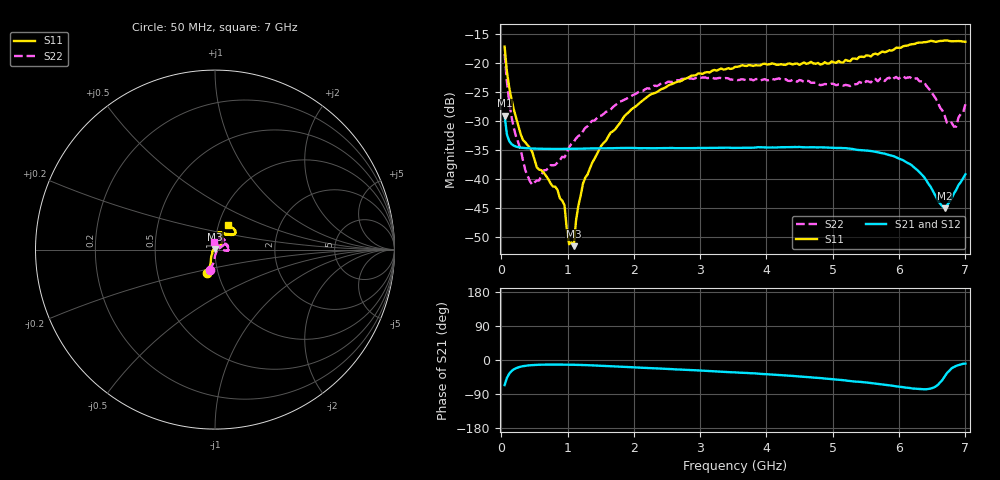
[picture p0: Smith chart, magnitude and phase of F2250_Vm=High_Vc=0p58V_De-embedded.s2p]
! Integrated Device Technology
! Corporate Headquarters
! 6024 Silver Creek Valley Road
! San Jose, CA 95138  USA
! Phone:  1-408-284-8200
! Toll Free:  1-800-223-1366
! Webpage:  http://www.idt.com/
! Timing and RF Division
! 515 Groton Road, Suite 102
! Westford, MA 01886-6024
! Device:  F2250
! Description: Voltage Variable RF Attenuator
! Frequency:  50.0 -  6000.00 MHz
! Package:  3x3 mm Thin QFN Plastic Package: 16 pin
! Ports:  2 RF, 3 DC
!  Pin  1  = GND
!  Pin  2  = NC
!  Pin  3  = RF1  = Port 1
!  Pin  4  = NC
!  Pin  5  = GND
!  Pin  6  = GND
!  Pin  7  = GND
!  Pin  8  = GND
!  Pin  9  = NC
!  Pin 10  = RF2  = Port 2
!  Pin 11  = NC
!  Pin 12  = GND
!  Pin 13  = GND
!  Pin 14  = VCNTRL
!  Pin 15  = VDD
!  Pin 16  = VMODE
! Vcntrl:  0.580 Volts
! Vmode:  +3.300 Volts
! Vdd:  +3.30  Volts
! Current:  1.276 mA
! Data:  The device was measured on a the F2250 evaluation board which has
!  individual transmission lines to the RF pins.  Data was collected
!  using a calibrated network analyzer.  The evaluation board was
!  de-embedded using a TRL calibration technique.
!  The reference plane is the edge of the package pin.
! Misc:  SN 10
!  Action Tracker AT0258
! Date Measured:  2014-11-26
! Date:  2015-10-15  MJV
! Note:
!  Integrated Device Technology supplies this data as a sample of measured
!  data at the package pin for this product.  Your particular data for this
!  product may vary.
!  Data was taken at 25 degrees C.
!  Integrated Device Technology reserves the right to change this data at anytime.
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# GHz S dB R 50
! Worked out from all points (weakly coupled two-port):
!   201 points, 50 MHz to 7 GHz, reference 50 ohm
!   highest |S21| = -29.07 dB at 50 MHz (marker M1); lowest = -45.0 dB at 6.687 GHz (marker M2)
!   lowest |S11| = -51.5 dB at 1.093 GHz (marker M3), VSWR 1.01, Z = 50 + j0.264 ohm
!   |S11| at or under -10 dB: start of sweep to end of sweep
!   |S22| runs from -41.0 to -18.4 dB; largest |S21 - S12| = 5.8e-05
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0.05  -17.17 -108.4  -29.07 -66.3  -29.07 -66.3  -18.43 -104.8
0.08475  -21.46 -107.2  -32.30 -47.3  -32.30 -47.3  -23.22 -94.7
0.189  -28.01 -119.7  -34.23 -24.7  -34.23 -24.7  -31.20 -85.5
0.328  -33.28 -133.6  -34.61 -16.3  -34.61 -16.3  -36.79 -56.9
0.467  -35.33 -145.7  -34.72 -13.5  -34.72 -13.4  -40.96 -27.2
0.5365  -37.98 -154.2  -34.75 -12.8  -34.75 -12.8  -40.25 -15.4
0.8145  -41.30 170.0  -34.80 -12.0  -34.80 -12.0  -37.54 13.2
0.9535  -44.51 171.1  -34.80 -12.2  -34.81 -12.2  -36.23 17.6
1.023  -51.20 139.0  -34.80 -12.4  -34.79 -12.4  -34.51 18.4
1.0925  -51.54 85.6  -34.78 -12.6  -34.78 -12.6  -33.58 20.2
1.12725  -47.13 58.7  -34.77 -12.7  -34.76 -12.8  -32.99 18.2
1.2315  -40.80 39.8  -34.74 -13.2  -34.74 -13.2  -31.76 16.6
1.6485  -31.99 40.8  -34.68 -16.2  -34.68 -16.2  -28.04 25.4
2.37825  -24.75 46.5  -34.65 -22.5  -34.66 -22.5  -23.79 33.6
3.525  -20.66 71.6  -34.61 -32.6  -34.61 -32.7  -22.85 60.6
4.7065  -20.07 71.9  -34.50 -46.3  -34.50 -46.3  -23.40 62.7
5.2625  -19.67 53.1  -34.74 -55.4  -34.73 -55.5  -23.97 40.6
5.85325  -17.80 40.5  -35.85 -66.8  -35.84 -67.0  -22.52 11.7
6.3745  -16.41 40.9  -39.60 -77.2  -39.61 -77.3  -23.21 -4.9
6.68725  -16.12 47.8  -45.00 -43.4  -45.00 -43.2  -29.05 16.7
6.861  -16.23 54.4  -41.85 -15.5  -41.81 -15.5  -30.95 59.8
7  -16.33 62.4  -39.16 -9.5  -39.14 -9.6  -27.10 94.0
